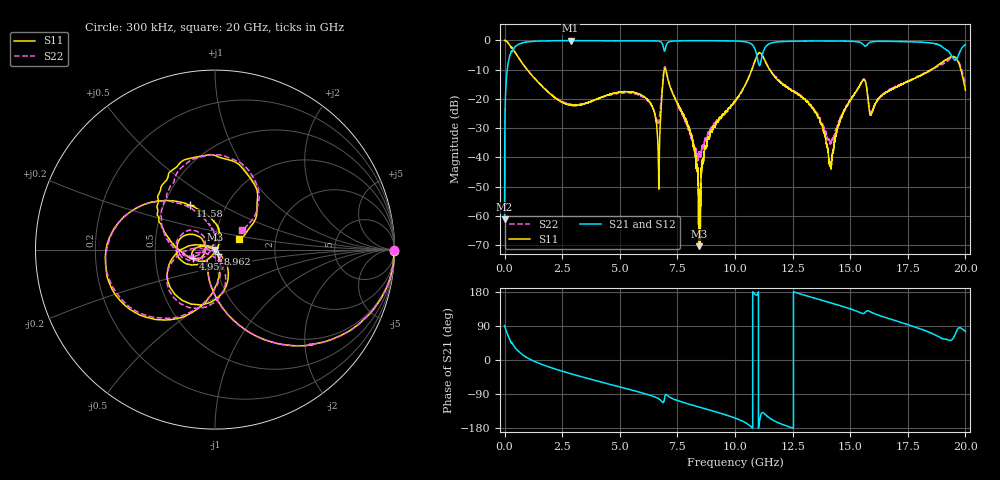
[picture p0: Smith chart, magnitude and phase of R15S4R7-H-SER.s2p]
!{R15S4R7}
!Johanson Technology Inc.
!www.johansontechnology.com
!Test Board Conditions:
!Substrate Type  RO4350B
!Substrate Thickness  20 mil
!Substrate Dk  3.66
!TL Type: GCPW
!TL Trace Width  34 mil
!TL Gap  10 mil
!Electrode orientation  Horizontal
!DUT TOPOLOGY	SERIES
!Mounting Pad LxW  26x52 mil
! Created Sat Feb  6 13:57:31 2021
# hz S ma R 50
! 2 Port Network Data from SP1.SP block
! freq  magS11  angS11  magS21  angS21  magS12  angS12  magS22  angS22
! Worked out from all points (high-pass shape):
!   20001 points, 300 kHz to 20 GHz, reference 50 ohm
!   highest |S21| = -0.05 dB at 2.861 GHz (marker M1); lowest = -61.2 dB at 300 kHz (marker M2)
!   |S21| within 3 dB of the highest: 366.5 MHz to 6.912 GHz (6.545 GHz wide, 180 % of centre); 11.27 GHz to 19.15 GHz (7.88 GHz wide, 51.8 % of centre)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
!   lowest |S11| = -70.3 dB at 8.435 GHz (marker M3), VSWR 1.00, Z = 50 - j0.0149 ohm
!   |S11| at or under -10 dB: 979.5 MHz to 6.928 GHz (5.949 GHz wide, 150 % of centre); 6.993 GHz to 10.73 GHz (3.735 GHz wide, 42.2 % of centre); 11.51 GHz to 18.51 GHz (7.003 GHz wide, 46.6 % of centre)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
!   |S22| runs from -41.2 to 0.0 dB; largest |S21 - S12| = 0.014
!   S11 on the Smith chart (normalised r, x): 300 kHz: open; 4.957 GHz: 0.78, -0.08; 8.962 GHz: 1.03, -0.05; 11.58 GHz: 0.68, +0.36; 20 GHz: 1.29, +0.15
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300000  1 -0.3  0.0008714 91.0  0.0009008 91.1  0.9985 -0.3
1.143e8  0.9476 -20.0  0.3156 69.7  0.3166 69.7  0.9464 -20.0
3.253e8  0.7463 -45.5  0.6593 44.2  0.6606 44.2  0.7478 -45.4
2.8613e9  0.07806 -123.5  0.9938 -35.9  0.9917 -35.9  0.08036 -128.2
3.3343e9  0.08021 -129.5  0.9911 -44.0  0.9902 -44.1  0.08188 -138.8
4.9573e9  0.1303 -157.6  0.9858 -70.4  0.9849 -70.4  0.1269 -162.5
6.2623e9  0.09204 170.6  0.9863 -92.1  0.9864 -92.0  0.08958 -169.2
6.6673e9  0.01166 164.3  0.9756 -101.7  0.9762 -101.6  0.03857 -117.8
6.9993e9  0.3092 -149.1  0.785 -90.8  0.7864 -90.7  0.3216 -146.5
8.0723e9  0.02644 146.5  0.9888 -117.8  0.9898 -117.7  0.02429 -172.7
8.4353e9  0.0003042 -150.6  0.9898 -124.1  0.9898 -124.1  0.01145 -106.9
8.9623e9  0.02818 -54.0  0.988 -133.2  0.9898 -133.3  0.03217 -52.5
1.00003e10  0.09171 -71.2  0.9781 -153.2  0.9777 -153.1  0.09107 -65.8
1.10293e10  0.6114 -156.5  0.3938 -176.6  0.3986 -176.6  0.6003 -157.2
1.15813e10  0.2824 119.5  0.9044 -156.5  0.9072 -156.6  0.2925 123.6
1.33343e10  0.07154 69.0  0.9789 165.4  0.9788 165.4  0.07533 92.4
1.41503e10  0.00739 -27.1  0.9797 150.8  0.9807 150.9  0.01726 156.9
1.55163e10  0.1982 -162.7  0.8855 123.0  0.8927 123.1  0.1984 -173.0
1.59113e10  0.05475 -176.1  0.9408 126.1  0.9428 126.2  0.05509 167.5
1.66673e10  0.1379 -158.4  0.9686 109.4  0.9599 109.3  0.1395 -164.5
1.94283e10  0.5267 101.6  0.5241 54.4  0.528 54.6  0.5209 100.2
2e10  0.1405 23.9  0.8488 75.4  0.8464 75.4  0.1823 35.9
